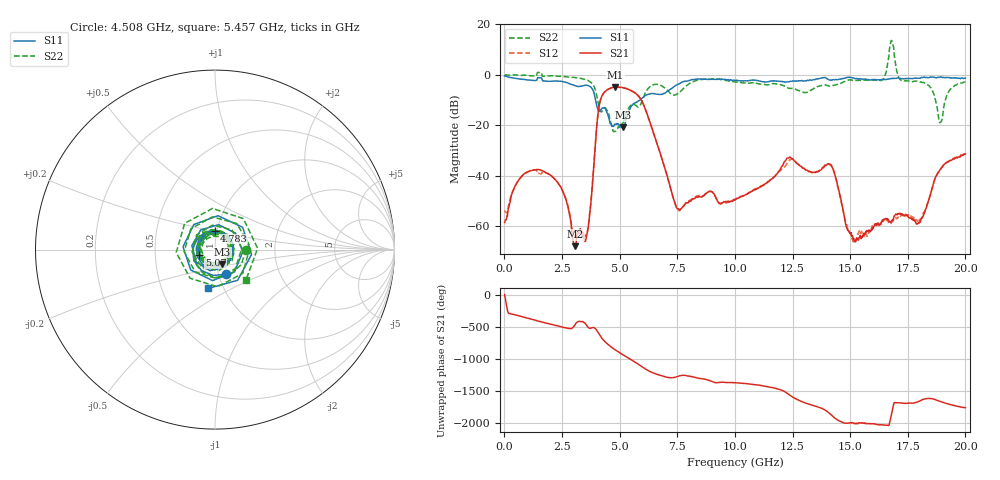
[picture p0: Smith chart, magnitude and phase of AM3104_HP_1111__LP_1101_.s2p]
!Created with skrf (http://scikit-rf.org).
# Hz S RI R 50.0
!freq ReS11 ImS11 ReS21 ImS21 ReS12 ImS12 ReS22 ImS22
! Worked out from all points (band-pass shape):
!   1601 points, 10 MHz to 20 GHz, reference 50 ohm
!   highest |S21| = -4.82 dB at 4.82 GHz (marker M1); lowest = -68.0 dB at 3.071 GHz (marker M2)
!   |S21| within 3 dB of the highest: 4.266 GHz to 5.759 GHz (1.493 GHz wide, 29.8 % of centre)
!   lowest |S11| = -20.9 dB at 5.145 GHz (marker M3), VSWR 1.20, Z = 53.6 - j8.71 ohm
!   |S11| at or under -10 dB: 3.954 GHz to 5.886 GHz (1.931 GHz wide, 39.3 % of centre)
!   |S22| runs from -22.6 to 13.6 dB; largest |S21 - S12| = 0.066
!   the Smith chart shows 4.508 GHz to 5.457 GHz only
!   S11 on the Smith chart (normalised r, x): 4.508 GHz: 1.09, -0.30; 4.783 GHz: 0.97, +0.21; 5.07 GHz: 0.84, -0.05; 5.457 GHz: 0.85, -0.39
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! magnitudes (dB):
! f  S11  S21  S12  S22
! 10 MHz  -0.4  -58.6  -53.8  0.0
! 1.572 GHz  -1.2  -37.8  -39.3  0.9
! 3.071 GHz  -4.3  -68.0  -64.4  -1.1
! 3.346 GHz  -4.5  -62.5  -62.2  -1.5
! 3.633 GHz  -4.3  -60.9  -60.8  -2.2
! 4.133 GHz  -14.5  -11.3  -11.4  -13.6
! 4.508 GHz  -16.5  -5.7  -5.8  -15.2
! 4.783 GHz  -19.5  -4.9  -4.9  -22.4
! 4.82 GHz  -19.7  -4.8  -4.9  -22.4
! 5.07 GHz  -20.8  -5.0  -5.0  -20.2
! 5.145 GHz  -20.9  -5.1  -5.1  -19.1
! 5.457 GHz  -13.2  -6.1  -6.1  -12.4
! 6.682 GHz  -7.8  -28.9  -29.0  -3.8
! 7.556 GHz  -3.6  -53.3  -53.5  -7.3
! 10.01 GHz  -2.3  -49.6  -49.4  -2.9
! 13.34 GHz  -2.1  -38.7  -38.7  -5.9
! 14.2 GHz  -2.1  -36.3  -36.5  -4.4
! 15.14 GHz  -1.3  -65.2  -66.2  -2.2
! 16.68 GHz  -1.6  -57.8  -58.5  7.3
! 17.98 GHz  -1.3  -58.8  -58.5  -2.7
! 18.91 GHz  -0.8  -37.5  -37.6  -18.9
! 20 GHz  -1.3  -31.4  -31.0  -2.8
